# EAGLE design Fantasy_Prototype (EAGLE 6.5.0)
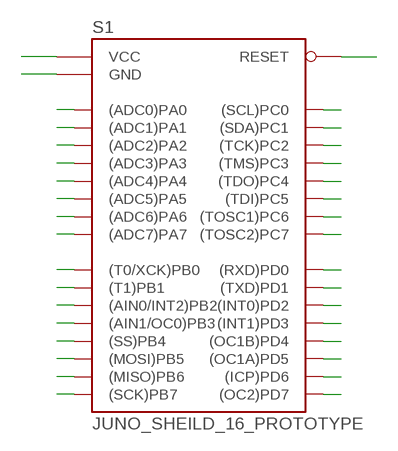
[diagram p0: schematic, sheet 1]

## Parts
S1  JUNO_SHEILD_16_PROTOTYPE  [JUNO_SHEILD_16_PROTOTYPE]

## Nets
N$5: S1.VCC1(VCC) S1.VCC2(VCC) S1.VCC3(VCC) S1.VCC4(VCC) S1.VCC5(VCC)
N$6: S1.GND1(GND) S1.GND2(GND) S1.GND3(GND) S1.GND4(GND) S1.GND5(GND) S1.GND6(GND)
N$7: S1.RST1(RESET) S1.RST2(RESET)
N$8: S1.A0((ADC0)PA0) S1.A0-((ADC0)PA0)
N$9: S1.A1((ADC1)PA1) S1.A1-((ADC1)PA1)
N$10: S1.A2((ADC2)PA2) S1.A2-((ADC2)PA2)
N$11: S1.A3((ADC3)PA3) S1.A3-((ADC3)PA3)
N$12: S1.A4((ADC4)PA4) S1.A4-((ADC4)PA4)
N$13: S1.A5((ADC5)PA5) S1.A5-((ADC5)PA5)
N$14: S1.A6((ADC6)PA6) S1.A6-((ADC6)PA6)
N$15: S1.A7((ADC7)PA7) S1.A7-((ADC7)PA7)
N$16: S1.B0((T0/XCK)PB0) S1.B0-((T0/XCK)PB0)
N$17: S1.B1((T1)PB1) S1.B1-((T1)PB1)
N$18: S1.B2((AIN0/INT2)PB2) S1.B2-((AIN0/INT2)PB2)
N$19: S1.B3((AIN1/OC0)PB3) S1.B3-((AIN1/OC0)PB3)
N$20: S1.B4((SS)PB4) S1.B4-((SS)PB4)
N$21: S1.B5((MOSI)PB5) S1.B5-((MOSI)PB5) S1.MOSI((MOSI)PB5)
N$22: S1.B6((MISO)PB6) S1.B6-((MISO)PB6) S1.MISO((MISO)PB6)
N$23: S1.B7((SCK)PB7) S1.B7-((SCK)PB7) S1.SCK((SCK)PB7)
N$24: S1.D7((OC2)PD7) S1.D7-((OC2)PD7)
N$25: S1.D6((ICP)PD6) S1.D6-((ICP)PD6)
N$26: S1.D5((OC1A)PD5) S1.D5-((OC1A)PD5)
N$27: S1.D4((OC1B)PD4) S1.D4-((OC1B)PD4)
N$28: S1.D3((INT1)PD3) S1.D3-((INT1)PD3)
N$29: S1.D2((INT0)PD2) S1.D2-((INT0)PD2)
N$30: S1.D1((TXD)PD1) S1.D1-((TXD)PD1)
N$31: S1.D0((RXD)PD0) S1.D0-((RXD)PD0)
N$32: S1.C7((TOSC2)PC7) S1.C7-((TOSC2)PC7)
N$33: S1.C0((SCL)PC0) S1.C0-((SCL)PC0)
N$34: S1.C1((SDA)PC1) S1.C1-((SDA)PC1)
N$35: S1.C2((TCK)PC2) S1.C2-((TCK)PC2)
N$36: S1.C3((TMS)PC3) S1.C3-((TMS)PC3)
N$37: S1.C4((TDO)PC4) S1.C4-((TDO)PC4)
N$38: S1.C5((TDI)PC5) S1.C5-((TDI)PC5)
N$39: S1.C6((TOSC1)PC6) S1.C6-((TOSC1)PC6)

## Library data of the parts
S1 = My Eagle lbr:JUNO_SHEILD_16_PROTOTYPE

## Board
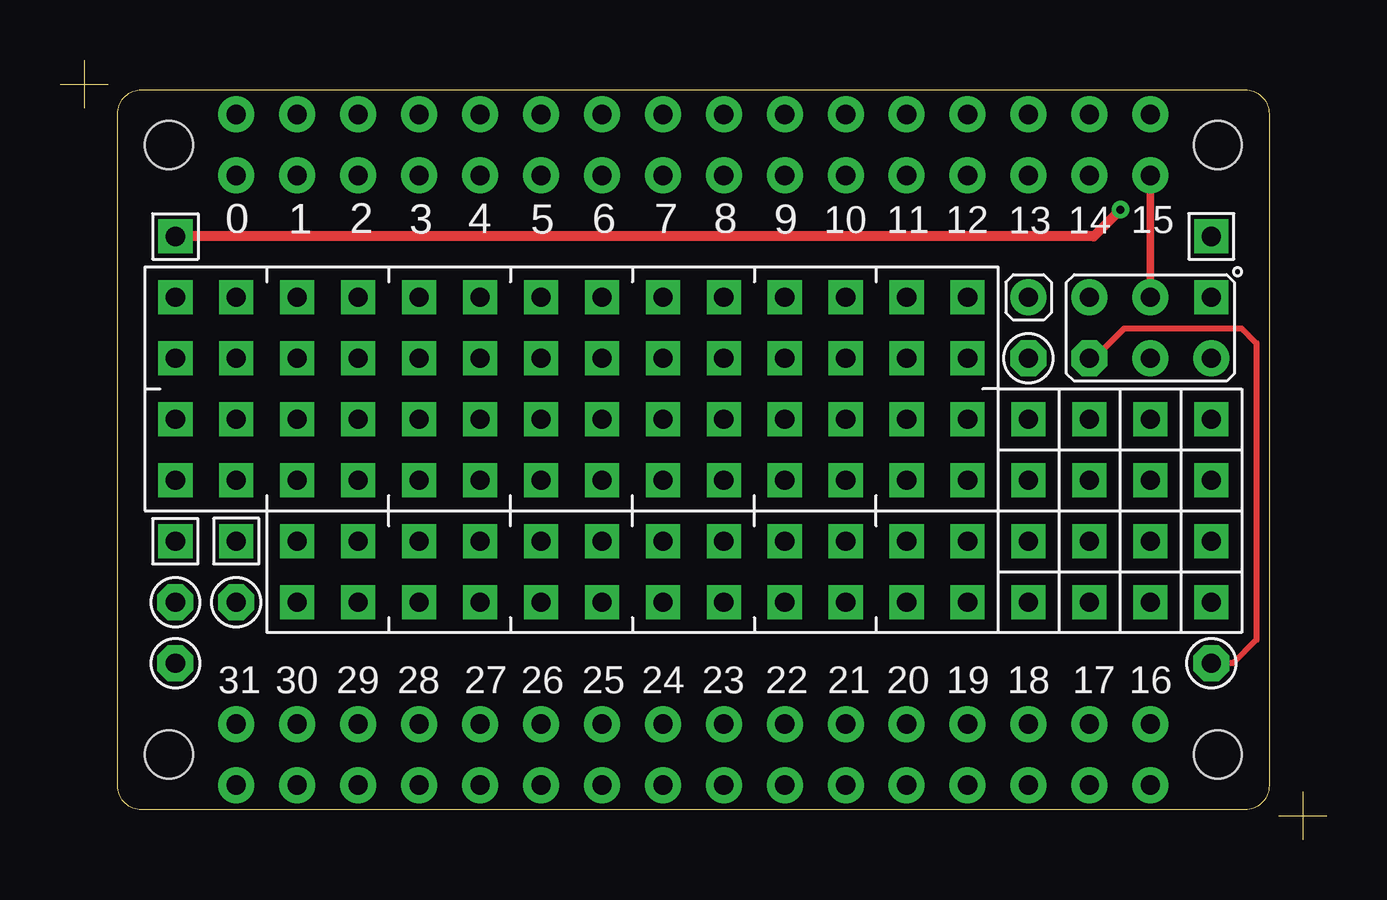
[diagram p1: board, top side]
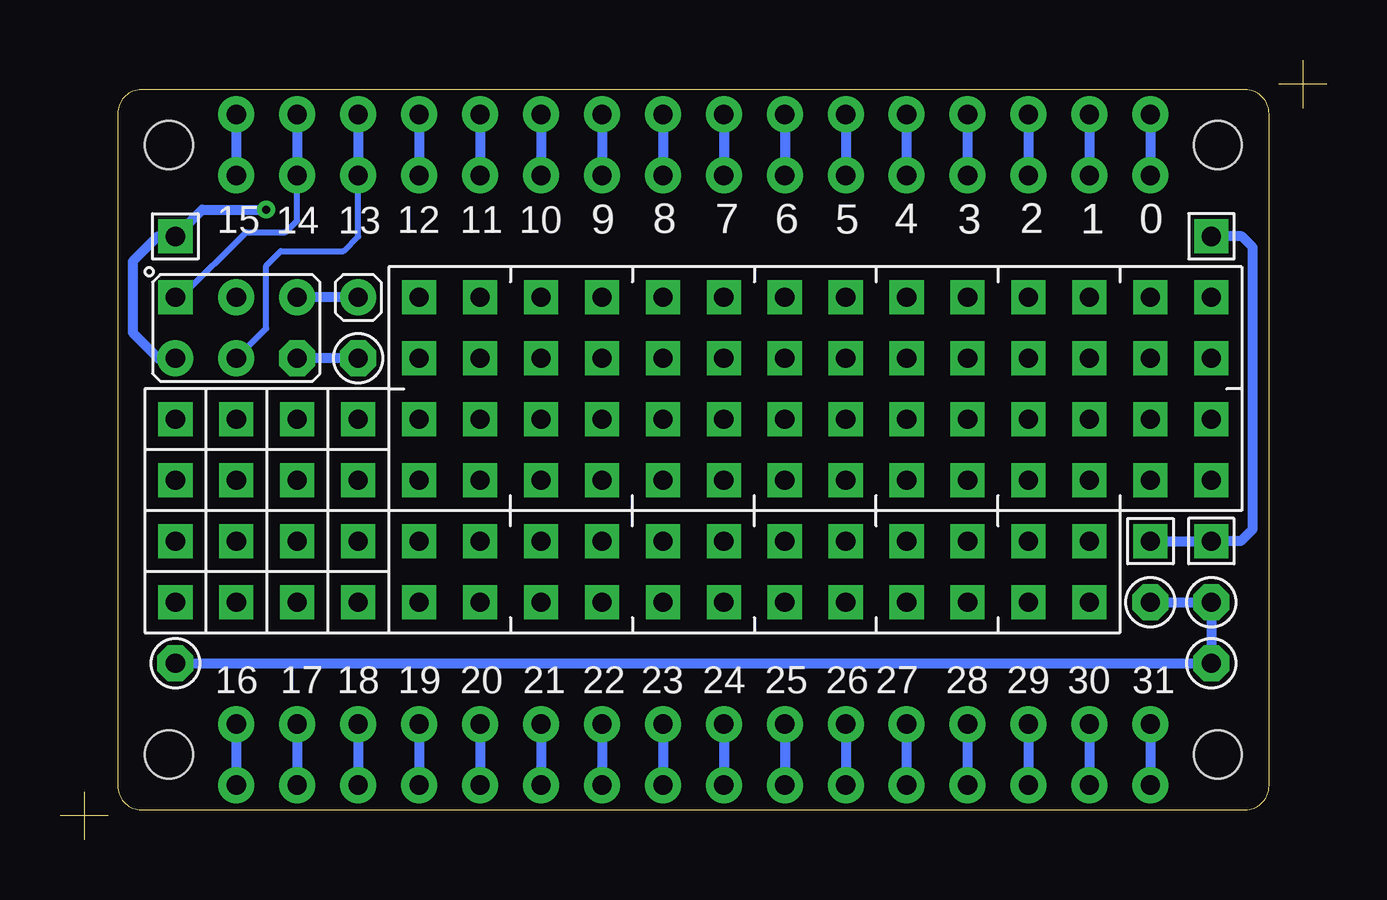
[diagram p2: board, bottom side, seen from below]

Size 52.8 x 32.48 mm. Coordinates in mm from the lower left corner, seen from the top.
Outline: 0,31.48 2,31.48
Outline: 1,32.48 1,30.48
Outline: 50.8,1 52.8,1
Outline: 51.8,2 51.8,0
Copper layers (1*16): Top 0.035mm / dielectric 1.5mm / Bottom 0.035mm
Design rules "10mm": minimum track width 10mil, minimum drill 0.3mm, track to track 6mil, track to pad 8mil, pad to pad 8mil, via to via 8mil, smd to smd 6mil, copper to edge 10mil, drill to drill 6mil, minimum pad ring 10mil, minimum via ring 8mil, stop-mask expansion 1mil, vias tented up to drill 0.4mm, thermal gap 10mil

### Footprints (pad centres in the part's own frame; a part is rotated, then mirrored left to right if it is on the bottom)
JUNO_SHEILD_16_PROTOTYPE = drill 0.8 pad 1.5: A0 -19.05,13.97; A0- -19.05,11.43; A1 -16.51,13.97; A1- -16.51,11.43; A2 -13.97,13.97; A2- -13.97,11.43; A3 -11.43,13.97; A3- -11.43,11.43; A4 -8.89,13.97; A4- -8.89,11.43; A5 -6.35,13.97; A5- -6.35,11.43; A6 -3.81,13.97; A6- -3.81,11.43; A7 -1.27,13.97; A7- -1.27,11.43; B0 1.27,13.97; B0- 1.27,11.43; B1 3.81,13.97; B1- 3.81,11.43; B2 6.35,13.97; B2- 6.35,11.43; B3 8.89,13.97; B3- 8.89,11.43; B4 11.43,13.97; B4- 11.43,11.43; B5 13.97,13.97; B5- 13.97,11.43; B6 16.51,13.97; B6- 16.51,11.43; B7 19.05,13.97; B7- 19.05,11.43; C0 19.05,-13.97; C0- 19.05,-11.43; C1 16.51,-13.97; C1- 16.51,-11.43; C2 13.97,-13.97; C2- 13.97,-11.43; C3 11.43,-13.97; C3- 11.43,-11.43; C4 8.89,-13.97; C4- 8.89,-11.43; C5 6.35,-13.97; C5- 6.35,-11.43; C6 3.81,-13.97; C6- 3.81,-11.43; C7 1.27,-13.97; C7- 1.27,-11.43; D0 -1.27,-13.97; D0- -1.27,-11.43; D1 -3.81,-13.97; D1- -3.81,-11.43; D2 -6.35,-13.97; D2- -6.35,-11.43; D3 -8.89,-13.97; D3- -8.89,-11.43; D4 -11.43,-13.97; D4- -11.43,-11.43; D5 -13.97,-13.97; D5- -13.97,-11.43; D6 -16.51,-13.97; D6- -16.51,-11.43; D7 -19.05,-13.97; D7- -19.05,-11.43; MOSI 19.05,3.81; RST1 16.51,6.35; RST2 13.97,6.35; SCK 19.05,6.35; VCC3 21.59,3.81 | drill 0.8 pad 1.5 octagon: GND1 -21.59,-6.35; GND2 -19.05,-6.35; GND3 16.51,3.81; GND4 13.97,3.81; GND5 -21.59,-8.89; GND6 21.59,-8.89 | drill 0.8 pad 1.422 square: MISO 21.59,6.35; P$1 -19.05,6.35; P$2 11.43,6.35; P$3 -13.97,3.81; P$4 -19.05,3.81; P$5 -19.05,1.27; P$6 -19.05,-1.27; P$7 -21.59,-1.27; P$8 -21.59,1.27; P$9 -21.59,3.81; P$10 -21.59,6.35; P$17 11.43,3.81; P$18 -16.51,-1.27; P$19 -13.97,-1.27; P$20 -11.43,-1.27; P$21 -8.89,-1.27; P$22 -6.35,-1.27; P$23 -3.81,-1.27; P$24 -1.27,-1.27; P$25 1.27,-1.27; P$26 3.81,-1.27; P$27 6.35,-1.27; P$28 8.89,-1.27; P$29 11.43,-1.27; P$30 11.43,1.27; P$38 -16.51,6.35; P$39 -16.51,3.81; P$40 -16.51,1.27; P$41 -13.97,6.35; P$43 -13.97,1.27; P$44 -11.43,6.35; P$45 -11.43,3.81; P$46 -11.43,1.27; P$47 -8.89,6.35; P$48 -8.89,3.81; P$49 -8.89,1.27; P$50 -6.35,6.35; P$51 -6.35,3.81; P$52 -6.35,1.27; P$53 -3.81,6.35; P$54 -3.81,3.81; P$55 -3.81,1.27; P$56 -1.27,6.35; P$57 -1.27,3.81; P$58 -1.27,1.27; P$59 1.27,6.35; P$60 1.27,3.81; P$61 1.27,1.27; P$62 3.81,6.35; P$63 3.81,3.81; P$64 3.81,1.27; P$65 6.35,6.35; P$66 6.35,3.81; P$67 6.35,1.27; P$68 8.89,6.35; P$69 8.89,3.81; P$70 8.89,1.27; P$71 13.97,1.27; P$72 16.51,1.27; P$73 19.05,1.27; P$74 21.59,1.27; P$75 13.97,-1.27; P$76 16.51,-1.27; P$77 19.05,-1.27; P$78 21.59,-1.27; P$79 -16.51,-3.81; P$80 -16.51,-6.35; P$82 -13.97,-3.81; P$83 -13.97,-6.35; P$85 -11.43,-3.81; P$86 -11.43,-6.35; P$88 -8.89,-3.81; P$89 -8.89,-6.35; P$91 -6.35,-3.81; P$92 -6.35,-6.35; P$94 -3.81,-3.81; P$95 -3.81,-6.35; P$97 -1.27,-3.81; P$98 -1.27,-6.35; P$100 1.27,-3.81; P$101 1.27,-6.35; P$103 3.81,-3.81; P$104 3.81,-6.35; P$106 6.35,-3.81; P$107 6.35,-6.35; P$109 8.89,-3.81; P$110 8.89,-6.35; P$112 11.43,-3.81; P$113 11.43,-6.35; P$115 13.97,-3.81; P$116 16.51,-3.81; P$117 19.05,-3.81; P$118 21.59,-3.81; P$119 21.59,-6.35; P$120 19.05,-6.35; P$121 16.51,-6.35; P$122 13.97,-6.35; VCC1 -21.59,-3.81; VCC2 -19.05,-3.81; VCC4 -21.59,8.89; VCC5 21.59,8.89 | hole 2: -21.86,12.7; 21.86,12.7; 21.86,-12.7; -21.86,-12.7

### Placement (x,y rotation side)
S1  26.4,16.24 0 top

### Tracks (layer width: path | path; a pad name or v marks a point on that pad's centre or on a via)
N$1
  Bottom 0: 0,31.48 2,31.48
N$2
  Top 0: 0,31.48 2,31.48
N$3
  Top 0: 1,32.48 1,30.48
N$4
  Bottom 0: 1,32.48 1,30.48
N$5  (via drill 0.33)
  Top 0.406: v44.2,26.25 43.09,25.13 S1.VCC4
  Bottom 0.406: S1.VCC2 S1.VCC1 3.59,12.43 3.08,12.94 3.08,24.67 3.54,25.13 S1.VCC4 | S1.VCC3 48.7,20.05 49.77,21.12 49.77,24.09 48.73,25.13 S1.VCC5 46.87,26.25 v44.2,26.25
N$6
  Top 0.254: S1.GND6 48.9,7.35 49.87,8.32 49.87,20.69 49.26,21.3 44.36,21.3 43.11,20.05 S1.GND3
  Bottom 0.406: S1.GND2 S1.GND1 S1.GND5 S1.GND6 | S1.GND4 S1.GND3
N$7
  Bottom 0.406: S1.RST2 S1.RST1
N$8
  Bottom 0.406: S1.A0 S1.A0-
N$9
  Bottom 0.406: S1.A1 S1.A1-
N$10
  Bottom 0.406: S1.A2 S1.A2-
N$11
  Bottom 0.406: S1.A3 S1.A3-
N$12
  Bottom 0.406: S1.A4 S1.A4-
N$13
  Bottom 0.406: S1.A5 S1.A5-
N$14
  Bottom 0.406: S1.A6 S1.A6-
N$15
  Bottom 0.406: S1.A7 S1.A7-
N$16
  Bottom 0.406: S1.B0 S1.B0-
N$17
  Bottom 0.406: S1.B1 S1.B1-
N$18
  Bottom 0.406: S1.B2 S1.B2-
N$19
  Bottom 0.406: S1.B3 S1.B3-
N$20
  Bottom 0.406: S1.B4 S1.B4-
N$21
  Bottom 0.254: S1.MOSI 44.2,21.3 44.2,23.91 43.6,24.52 40.98,24.52 40.37,25.13 S1.B5-
  Bottom 0.305: S1.B5- 40.39,27.65
  Bottom 0.406: S1.B5 S1.B5-
N$22
  Bottom 0.254: S1.MISO 47.76,22.59 45.04,25.31 43.39,25.31 42.91,25.79 S1.B6-
  Bottom 0.305: S1.B6- 42.94,27.65
  Bottom 0.406: S1.B6 S1.B6-
N$23
  Top 0.305: S1.B7- S1.SCK
  Bottom 0.406: S1.B7 S1.B7-
N$24
  Bottom 0.406: S1.D7- S1.D7
N$25
  Bottom 0.406: S1.D6- S1.D6
N$26
  Bottom 0.406: S1.D5- S1.D5
N$27
  Bottom 0.406: S1.D4- S1.D4
N$28
  Bottom 0.406: S1.D3- S1.D3
N$29
  Bottom 0.406: S1.D2- S1.D2
N$30
  Bottom 0.406: S1.D1- S1.D1
N$31
  Bottom 0.406: S1.D0- S1.D0
N$32
  Bottom 0.406: S1.C7- S1.C7
N$33
  Bottom 0.406: S1.C0- S1.C0
N$34
  Bottom 0.406: S1.C1- S1.C1
N$35
  Bottom 0.406: S1.C2- S1.C2
N$36
  Bottom 0.406: S1.C3- S1.C3
N$37
  Bottom 0.406: S1.C4- S1.C4
N$38
  Bottom 0.406: S1.C5- S1.C5
N$39
  Bottom 0.406: S1.C6- S1.C6
N$40
  Top 0: 50.8,1 52.8,1
N$41
  Top 0: 51.8,2 51.8,0
N$42
  Bottom 0: 50.8,1 52.8,1
N$43
  Bottom 0: 51.8,2 51.8,0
